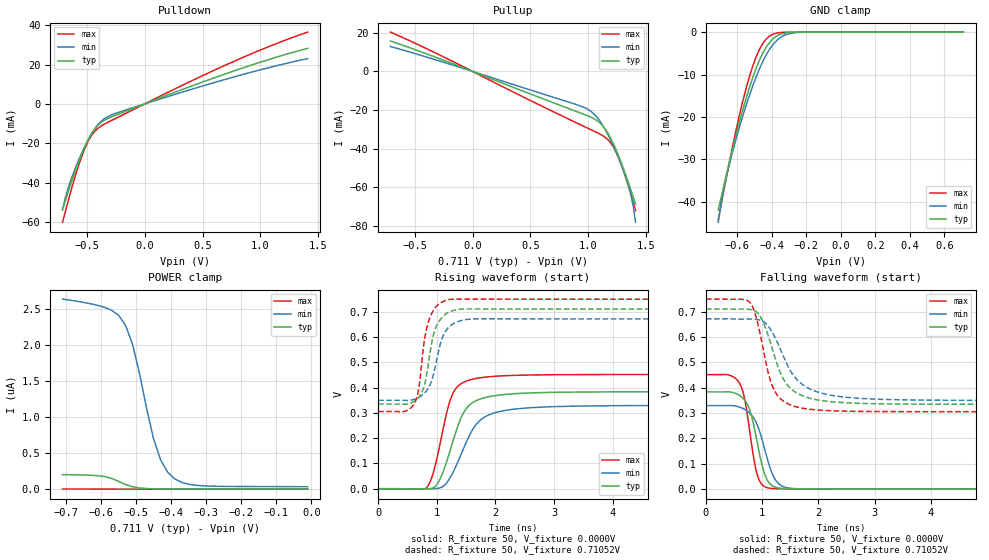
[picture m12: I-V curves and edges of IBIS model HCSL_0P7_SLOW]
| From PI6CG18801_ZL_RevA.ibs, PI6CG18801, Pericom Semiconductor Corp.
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[Model]   HCSL_0P7_SLOW
Model_type Output
Vref=0.7000V
Vmeas=900mV
| variable   typ   min   max
C_comp   2.000pF   1.970pF   2.030pF
[Voltage Range]   0.71052V   0.67147V   0.74949V
[POWER Clamp Reference]   0.71052V   0.67147V   0.74949V
[GND Clamp Reference]   0.0000V   0.0000V   0.0000V
[Pullup Reference]   0.71052V   0.67147V   0.74949V
[Pulldown Reference]   0.0000V   0.0000V   0.0000V
[Temperature Range]   25   85   -40
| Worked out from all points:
|   slope of the pulldown table from 0 to 0.107 V, typ, clamps not added: 43.9 ohm
|   slope of the pullup table from 0 to 0.107 V, typ, clamps not added: 42.4 ohm
|   GND clamp passes 1 mA (typ) near -0.37 V on its own axis
|   falling waveform, R_fixture 50, V_fixture 0.0000V: 20-80 % time 234ps typ, 279ps min, 194ps max; typ from 0.384 V to 0 V
|   rising waveform, R_fixture 50, V_fixture 0.0000V: 20-80 % time 350ps typ, 429ps min, 274ps max; typ from 0 V to 0.384 V
|   falling waveform, R_fixture 50, V_fixture 0.71052V: 20-80 % time 393ps typ, 501ps min, 294ps max; typ from 0.711 V to 0.335 V
|   rising waveform, R_fixture 50, V_fixture 0.71052V: 20-80 % time 191ps typ, 222ps min, 169ps max; typ from 0.335 V to 0.711 V
[GND Clamp]
| Voltage   I(typ)   I(min)   I(max)
-710.5mV  -41.93mA   -44.79mA   -44.29mA
-690.5mV  -38.38mA   -39.63mA   -39.99mA
-650.5mV  -31.43mA   -31.94mA   -31.6mA
-590.5mV  -21.65mA   -22.79mA   -20.07mA
-550.5mV  -15.81mA   -17.46mA   -13.46mA
-510.5mV  -10.7mA    -12.68mA   -8.013mA
-470.5mV  -6.503mA   -8.547mA   -3.986mA
-450.5mV  -4.807mA   -6.77mA    -2.569mA
-410.5mV  -2.292mA   -3.877mA   -863uA
-350.5mV  -515.2uA   -1.274mA   -104.6uA
-250.5mV  -20.58uA   -103.2uA   -1.252uA
709.5mV   1.155nA    34.32nA    -1.818pA
[POWER Clamp]
| Voltage   I(typ)   I(min)   I(max)
-710.5mV  202.2nA    2.638uA    2.798nA
-570.5mV  149.4nA    2.483uA    234pA
-550.5mV  108.7nA    2.413uA    105.5pA
-530.5mV  64.8nA     2.273uA    56.58pA
-510.5mV  33.41nA    2.008uA    37.69pA
-490.5mV  16.56nA    1.601uA    30.01pA
-450.5mV  4.682nA    697nA      24.52pA
-430.5mV  2.929nA    406.3nA    23.13pA
-410.5mV  2.112nA    236.4nA    21.95pA
-390.5mV  1.728nA    143.6nA    20.85pA
-310.5mV  1.373nA    46.52nA    16.62pA
-10.52mV  1.163nA    33.88nA    840fA
[Pulldown]
| Voltage   I(typ)   I(min)   I(max)
-710.5mV  -53.57mA   -53.89mA   -60.08mA
-690.5mV  -49.91mA   -48.65mA   -55.62mA
-650.5mV  -42.7mA    -40.76mA   -46.88mA
-550.5mV  -26.33mA   -25.71mA   -27.7mA
-510.5mV  -20.85mA   -20.65mA   -21.72mA
-470.5mV  -16.23mA   -16.21mA   -17.05mA
-410.5mV  -11.21mA   -10.96mA   -12.68mA
-350.5mV  -8.379mA   -7.605mA   -10.34mA
-290.5mV  -6.678mA   -5.686mA   -8.527mA
69.48mV   1.588mA    1.304mA    2.051mA
809.5mV   17.48mA    14.31mA    22.58mA
1.409V    28.24mA    23mA       36.47mA
[Pullup]
| Voltage   I(typ)   I(min)   I(max)
-710.5mV  15.78mA    12.92mA    20.39mA
869.5mV   -20.11mA   -16.62mA   -25.8mA
1.029V    -23.88mA   -20.96mA   -30.35mA
1.069V    -25.19mA   -23.25mA   -31.49mA
1.129V    -28.46mA   -28.28mA   -33.44mA
1.189V    -34.06mA   -35.02mA   -36.69mA
1.229V    -39.02mA   -40.24mA   -40.46mA
1.289V    -47.89mA   -49.02mA   -48.79mA
1.349V    -57.98mA   -59.53mA   -59.62mA
1.369V    -61.53mA   -64.06mA   -63.63mA
1.389V    -65.14mA   -69.88mA   -67.8mA
1.409V    -68.79mA   -78.13mA   -72.1mA
[Falling Waveform]
R_fixture = 50
V_fixture = 0.0000V
V_fixture_min = 0.0000V
V_fixture_max = 0.0000V
|   Time   V(typ)   V(min)   V(max)
0s        383.5mV    329.4mV    451.7mV
420ps     383.6mV    329.6mV    449.3mV
600ps     369.3mV    323.1mV    416.4mV
675ps     354.7mV    316.2mV    369.4mV
765ps     320.3mV    302.6mV    250.1mV
900ps     198.9mV    260mV      67.58mV
1.065ns   47.7mV     141.5mV    7.624mV
1.23ns    8.046mV    39.16mV    2.168mV
1.47ns    1.805mV    4.621mV    1.14mV
5ns       25.46uV    36.05uV    20.3uV
[Rising Waveform]
R_fixture = 50
V_fixture = 0.0000V
V_fixture_min = 0.0000V
V_fixture_max = 0.0000V
|   Time   V(typ)   V(min)   V(max)
0s        9.383uV    10.13uV    9.384uV
840ps     -134.3uV   -143.6uV   7.949mV
940ps     3.432mV    308.6uV    62.18mV
1.04ns    31.36mV    2.544mV    159.6mV
1.26ns    175.2mV    57.31mV    369.2mV
1.46ns    301.7mV    160.8mV    421.1mV
1.66ns    346.8mV    250.6mV    435.5mV
2ns       368.2mV    300.9mV    444.8mV
2.8ns     380.2mV    322.8mV    450.4mV
10ns      383.5mV    329.4mV    451.7mV
[Falling Waveform]
R_fixture = 50
V_fixture = 0.71052V
V_fixture_min = 0.67147V
V_fixture_max = 0.74949V
|   Time   V(typ)   V(min)   V(max)
0s        710.5mV    671.5mV    749.5mV
780ps     708.6mV    670.7mV    736.5mV
880ps     701.9mV    669.5mV    687.8mV
980ps     675.5mV    665.1mV    595.4mV
1.2ns     539.1mV    610.7mV    397.4mV
1.4ns     426mV      513.2mV    343.8mV
1.68ns    372mV      419.2mV    320.8mV
2.1ns     348mV      376.3mV    310.5mV
3ns       337mV      355.1mV    306.2mV
10ns      334.6mV    349.7mV    305.4mV
[Rising Waveform]
R_fixture = 50
V_fixture = 0.71052V
V_fixture_min = 0.67147V
V_fixture_max = 0.74949V
|   Time   V(typ)   V(min)   V(max)
0s        334.6mV    349.7mV    305.4mV
445ps     333.9mV    349.6mV    305.7mV
610ps     345.3mV    353.1mV    334.1mV
685ps     360.1mV    360.4mV    385.3mV
790ps     409.8mV    378.3mV    587.7mV
850ps     483.1mV    395.7mV    653.4mV
970ps     628.7mV    477.6mV    714.1mV
1.135ns   687.5mV    617.1mV    743.3mV
1.6ns     711.2mV    671.2mV    749.9mV
5ns       710.5mV    671.5mV    749.5mV
[Ramp]
| variable   typ   min   max
dV/dt_r   0.23027V/349.47p   0.19779V/428.73p   0.27126V/273.87p
dV/dt_f   0.22544V/392.27p   0.19310V/500.97p   0.26632V/293.49p
R_load = 50
